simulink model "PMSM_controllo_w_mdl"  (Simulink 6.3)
settings: Solver=ode45  StartTime=0.0  StopTime=12.0  RelTol=1e-3
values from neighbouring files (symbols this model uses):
  bm = 0.8*N*metri*secondo/rad    (= 0.8)    [architetture_epicicloidale.m]    (also in architetture_epicicloidale_cont.m; architetture_epicicloidale_HEV.m; architetture_epicicloidale_prova.m; architetture_HEV_controllo.m)
  I_m = eye(m-1)    [architetture_epicicloidale.m]    (also in architetture_epicicloidale_cont.m; architetture_epicicloidale_HEV.m; architetture_epicicloidale_prova.m; architetture_HEV_controllo.m)
  Iw0 = 0*wI0    [architetture_epicicloidale.m]    (also in architetture_epicicloidale_cont.m = wI0; architetture_epicicloidale_HEV.m; architetture_epicicloidale_prova.m; architetture_HEV_controllo.m)
  Jm = 1.6*kg*metri^2    (= 1.6)    [architetture_epicicloidale.m]    (also in architetture_epicicloidale_cont.m; architetture_epicicloidale_HEV.m = 1.64945909552; architetture_epicicloidale_prova.m; architetture_HEV_controllo.m = 0.529459095518)
  Jr = Jr([1:m-1],[1:m-1])    [architetture_epicicloidale.m]    (also in architetture_epicicloidale_cont.m; architetture_epicicloidale_HEV.m; architetture_epicicloidale_prova.m; architetture_HEV_controllo.m)
  Kf = diag(diag(MLb)'./fliplr(tau_m(1:m-1)))    [architetture_epicicloidale_cont.m]    (also in architetture_epicicloidale_HEV.m; architetture_epicicloidale_prova.m; architetture_HEV_controllo.m; architetture_HEV_startstop.m)
  Kprop = 32.3*5    (= 161.5)    [architetture_HEV_controllo.m]    (also in architetture_HEV_startstop.m; PMSM_controllo_w.m = 32.3; architetture_HEV_startstop_1.m; architetture_HEV_startstop_2.m)
  Kr = Kr([1:m-1])    [architetture_epicicloidale.m]    (also in architetture_epicicloidale_cont.m; architetture_epicicloidale_HEV.m; architetture_epicicloidale_prova.m; architetture_HEV_controllo.m)
  Li = 0.1*Henry    (= 0.1)    [architetture_epicicloidale.m]    (also in architetture_epicicloidale_cont.m; architetture_epicicloidale_HEV.m; architetture_epicicloidale_prova.m; architetture_HEV_controllo.m)
  m = 5    [architetture_epicicloidale.m]    (also in architetture_epicicloidale_cont.m; architetture_epicicloidale_HEV.m; architetture_epicicloidale_prova.m; architetture_HEV_controllo.m)
  Mi = 0.08*Henry    (= 0.08)    [architetture_epicicloidale.m]    (also in architetture_epicicloidale_cont.m; architetture_epicicloidale_HEV.m; architetture_epicicloidale_prova.m; architetture_HEV_controllo.m)
  MKr = MKr([1:m-1],[1:m-1])    [architetture_epicicloidale.m]    (also in architetture_epicicloidale_cont.m; architetture_epicicloidale_HEV.m; architetture_epicicloidale_prova.m; architetture_HEV_controllo.m)
  MLb = MLb([1:m-1],[1:m-1])    [architetture_epicicloidale.m]    (also in architetture_epicicloidale_cont.m; architetture_epicicloidale_HEV.m; architetture_epicicloidale_prova.m; architetture_HEV_controllo.m)
  MR = MR([1:m-1],[1:m-1])    [architetture_epicicloidale.m]    (also in architetture_epicicloidale_cont.m; architetture_epicicloidale_HEV.m; architetture_epicicloidale_prova.m; architetture_HEV_controllo.m)
  Nar = 200    [architetture_epicicloidale.m]    (also in architetture_epicicloidale_cont.m; architetture_epicicloidale_HEV.m; architetture_epicicloidale_prova.m; architetture_HEV_controllo.m)
  Nc = 30    [architetture_epicicloidale.m]    (also in architetture_epicicloidale_cont.m; architetture_epicicloidale_HEV.m; architetture_epicicloidale_prova.m; architetture_HEV_controllo.m)
  p = 1    [architetture_epicicloidale.m]    (also in architetture_epicicloidale_cont.m; architetture_epicicloidale_HEV.m; architetture_epicicloidale_prova.m; architetture_HEV_controllo.m)
  Phir = 0.02*Weber    (= 0.02)    [architetture_epicicloidale.m]    (also in architetture_epicicloidale_cont.m; architetture_epicicloidale_HEV.m; architetture_epicicloidale_prova.m; architetture_HEV_controllo.m)
  Ri = 3*Ohm    (= 3)    [architetture_epicicloidale.m]    (also in architetture_epicicloidale_cont.m; architetture_epicicloidale_HEV.m; architetture_epicicloidale_prova.m; architetture_HEV_controllo.m = 0.1)
  Star = Si    [architetture_epicicloidale.m]    (also in architetture_epicicloidale_cont.m; architetture_epicicloidale_HEV.m; architetture_epicicloidale_prova.m; architetture_HEV_controllo.m)
  Tc = 0.05*ms    (= 5e-05)    [architetture_epicicloidale.m]    (also in architetture_epicicloidale_cont.m; architetture_epicicloidale_HEV.m; architetture_epicicloidale_prova.m; architetture_HEV_controllo.m)
  Tder = 0.0119*20    (= 0.238)    [architetture_HEV_controllo.m]    (also in architetture_HEV_startstop.m; PMSM_controllo_w.m; architetture_HEV_startstop_1.m; architetture_HEV_startstop_2.m)
  Thm0 = 0    [architetture_epicicloidale.m]    (also in architetture_epicicloidale_cont.m; architetture_epicicloidale_HEV.m; architetture_epicicloidale_prova.m; architetture_HEV_controllo.m)
  Tint = 0.2427*10    (= 2.427)    [architetture_HEV_controllo.m]    (also in architetture_HEV_startstop.m; PMSM_controllo_w.m = 0.2427; architetture_HEV_startstop_1.m; architetture_HEV_startstop_2.m)
  tTb = tTb(:,[1:m-1])    [architetture_epicicloidale.m]    (also in architetture_epicicloidale_cont.m; architetture_epicicloidale_HEV.m; architetture_epicicloidale_prova.m; architetture_HEV_controllo.m)
  Wm0 = 0*Wr_d    (= 0)    [architetture_epicicloidale.m]    (also in architetture_epicicloidale_cont.m = 62.5; architetture_epicicloidale_HEV.m; architetture_epicicloidale_prova.m; architetture_HEV_controllo.m)
libraries: simulink x2, POG_Sincronous_Motors x1

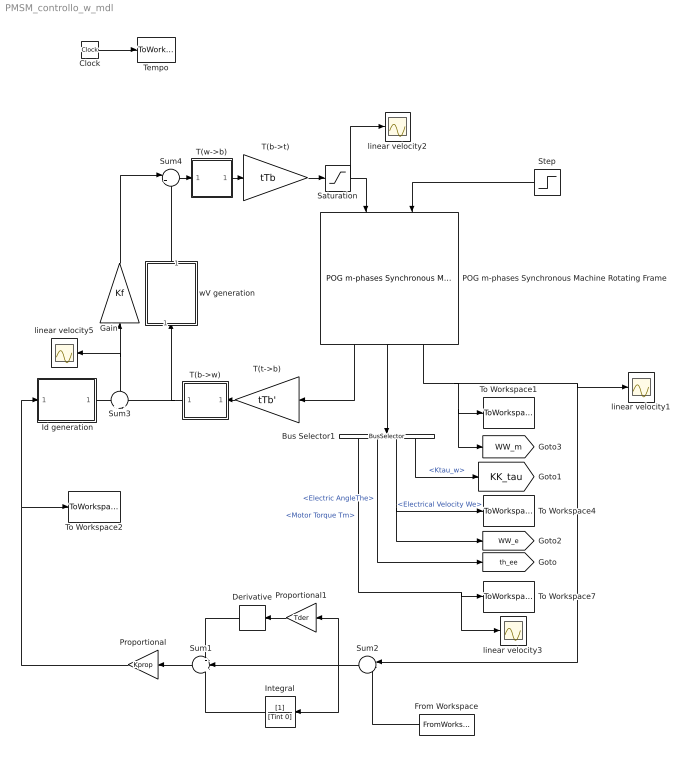
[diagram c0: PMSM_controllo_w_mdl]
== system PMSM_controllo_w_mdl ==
  " Id generation" : Subsystem
  Bus Selector1 : BusSelector  Orientation=down  OutputSignals=Motor Torque Tm,Electric AngleThe,Electrical Velocity We,Ktau_w
  Clock : Clock
  Derivative : Derivative  Orientation=left
  From Workspace : FromWorkspace  Orientation=left  VariableName=[T_in w_des]  SampleTime=0
  Gain : Gain  Orientation=up  Gain=Kf  Multiplication=Matrix(K*u) (u vector)
  Integral : TransferFcn  Orientation=left  Denominator=[Tint 0]
  POG m-phases Synchronous Machine Rotating Frame : POG_Sincronous_Motors/POG m-phases Synchronous Machine Rotating Frame  Orientation=down  Motor_Par=[m p]  Phase_Par=[Nc Star]  Electric_Par=[Ri Li Mi]  Mech_Par=[Jm bm]  Plux_Par=[Phir Nar]  Iniz_Cond=[Wm0; Thm0; Iw0]  TipoFlux=User defined  Tipo=Tipo  alfa=al  degree=6  TipoF=Tipo
  Proportional : Gain  Orientation=left  Gain=Kprop
  Proportional1 : Gain  Orientation=left  Gain=Tder
  Saturation : Saturate  UpperLimit=200  LowerLimit=-200
  Step : Step  Orientation=left  Time=5  After=100  SampleTime=0
  Sum1 : Sum  Orientation=left  Inputs=+++
  Sum2 : Sum  Orientation=left  Inputs=|-+
  Sum3 : Sum  Orientation=up  Inputs=+|-
  Sum4 : Sum  Inputs=|++
  T(b->t) : Gain  Gain=tTb  Multiplication=Matrix(K*u) (u vector)
  T(b->w) : Subsystem  Orientation=left  AncestorBlock=|
      | POG_Electric_Bloks/POG m-phases
      | Synchronous Machine
      | Rotating Frame/T(b->w)
  T(t->b) : Gain  Orientation=left  Gain=tTb'  Multiplication=Matrix(K*u) (u vector)
  T(w->b) : Subsystem  AncestorBlock=|
      | POG_Electric_Bloks/POG m-phases
      | Synchronous Machine
      | Rotating Frame/T(w->b)
  Tempo : ToWorkspace  VariableName=t  SampleTime=Tc  SaveFormat=Array
  To Workspace1 : ToWorkspace  VariableName=Wm  SampleTime=Tc  SaveFormat=Array
  To Workspace2 : ToWorkspace  VariableName=Tref  SampleTime=Tc  SaveFormat=Array
  To Workspace4 : ToWorkspace  VariableName=We  SampleTime=Tc  SaveFormat=Array
  To Workspace7 : ToWorkspace  VariableName=Tm  SampleTime=Tc  SaveFormat=Array
  linear velocity{1..3,5} (4 alike) : Scope
  wV generation : Subsystem  Orientation=up
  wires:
  Clock/1 -> Tempo/1
  POG m-phases Synchronous Machine Rotating Frame/3 -> To Workspace1/1, [WW_m], Sum2/1, linear velocity1/1
  POG m-phases Synchronous Machine Rotating Frame/2 -> Bus Selector1/1
  Bus Selector1/3 -> To Workspace4/1, [WW_e]  "<Electrical Velocity We>"
  T(w->b)/1(It) -> T(b->t)/1
  T(b->t)/1 -> Saturation/1
  T(t->b)/1 -> T(b->w)/1(Vt)
  T(b->w)/1(Vw) -> wV generation/1(In1), Sum3/2
  POG m-phases Synchronous Machine Rotating Frame/1 -> T(t->b)/1
  Bus Selector1/2 -> [th_ee]  "<Electric AngleThe>"
  Bus Selector1/1 -> To Workspace7/1, linear velocity3/1  "<Motor Torque Tm>"
  " Id generation"/1(Out1) -> Sum3/1
  Sum3/1 -> Gain/1, linear velocity5/1
  Sum4/1 -> T(w->b)/1(Iw)
  Gain/1 -> Sum4/1
  wV generation/1(Out1) -> Sum4/2
  Bus Selector1/4 -> [KK_tau]  "<Ktau_w>"
  Step/1 -> POG m-phases Synchronous Machine Rotating Frame/2
  Sum2/1 -> Integral/1, Proportional1/1, Sum1/2
  From Workspace/1 -> Sum2/2
  Sum1/1 -> Proportional/1
  Proportional1/1 -> Derivative/1
  Derivative/1 -> Sum1/1
  Integral/1 -> Sum1/3
  Proportional/1 -> " Id generation"/1(In1), To Workspace2/1
  Saturation/1 -> POG m-phases Synchronous Machine Rotating Frame/1, linear velocity2/1

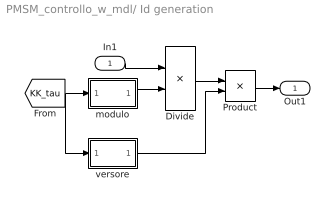
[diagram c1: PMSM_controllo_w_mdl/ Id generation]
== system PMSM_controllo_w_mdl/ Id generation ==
  In1 : Inport
  Divide : Product  Inputs=*/  OutScaling=2^-10
  Product : Product
  modulo : Subsystem
  versore : Subsystem
  Out1 : Outport
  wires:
  [KK_tau] -> modulo/1(In1), versore/1(In1)
  modulo/1(Out1) -> Divide/2
  Divide/1 -> Product/1
  versore/1(Out1) -> Product/2
  In1/1 -> Divide/1
  Product/1 -> Out1/1

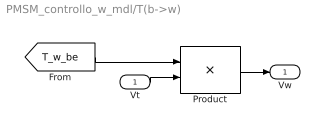
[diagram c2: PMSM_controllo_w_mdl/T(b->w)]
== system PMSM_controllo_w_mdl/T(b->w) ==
  Vt : Inport
  Product : Product  Multiplication=Matrix(*)
  Vw : Outport
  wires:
  Vt/1 -> Product/2
  Product/1 -> Vw/1
  [T_w_be] -> Product/1

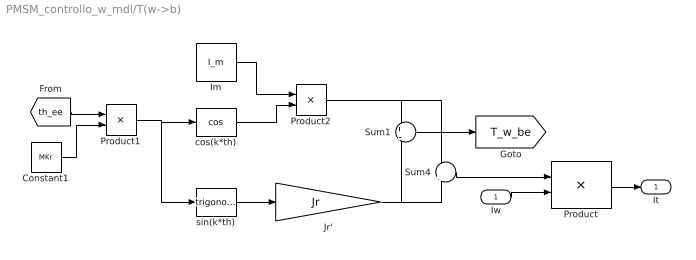
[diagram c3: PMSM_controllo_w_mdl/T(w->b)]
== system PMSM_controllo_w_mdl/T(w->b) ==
  Iw : Inport
  Constant1 : Constant  Value=MKr
  Im : Constant  Value=I_m  VectorParams1D=off
  Jr' : Gain  Gain=Jr  Multiplication=Matrix(K*u)
  Product : Product  Multiplication=Matrix(*)
  Product1 : Product
  Product2 : Product
  Sum1 : Sum  Inputs=+|-
  Sum4 : Sum  Inputs=+|+
  cos(k*th) : Trigonometry  Operator=cos
  sin(k*th) : Trigonometry
  It : Outport
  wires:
  Sum4/1 -> Product/1
  Product/1 -> It/1
  Iw/1 -> Product/2
  Jr'/1 -> Sum4/2, Sum1/2
  Product2/1 -> Sum4/1, Sum1/1
  Im/1 -> Product2/1
  cos(k*th)/1 -> Product2/2
  Product1/1 -> sin(k*th)/1, cos(k*th)/1
  Constant1/1 -> Product1/2
  [th_ee] -> Product1/1
  sin(k*th)/1 -> Jr'/1
  Sum1/1 -> [T_w_be]

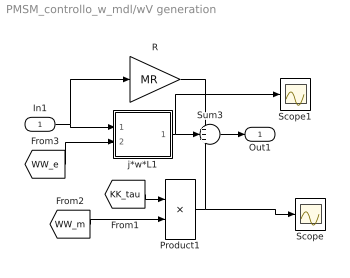
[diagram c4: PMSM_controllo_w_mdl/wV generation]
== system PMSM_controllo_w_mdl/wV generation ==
  In1 : Inport
  Product1 : Product  Multiplication=Matrix(*)
  R : Gain  Gain=MR  Multiplication=Matrix(K*u) (u vector)
  Scope : Scope
  Scope1 : Scope
  Sum3 : Sum  Inputs=+++
  j*w*L1 : Subsystem  AncestorBlock=|
      | POG_Electric_Bloks/POG m-phases
      | Synchronous Machine
      | Rotating Frame/j*w*L
  Out1 : Outport
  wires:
  [KK_tau] -> Product1/1
  [WW_m] -> Product1/2
  R/1 -> Sum3/1
  j*w*L1/1(Out1) -> Sum3/2, Scope1/1
  Product1/1 -> Sum3/3, Scope/1
  In1/1 -> j*w*L1/1(In1), R/1
  Sum3/1 -> Out1/1
  [WW_e] -> j*w*L1/2(In2)

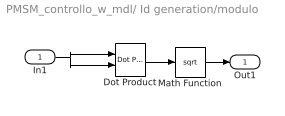
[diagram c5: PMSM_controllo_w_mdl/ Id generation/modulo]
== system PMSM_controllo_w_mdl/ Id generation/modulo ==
  In1 : Inport
  Dot Product : simulink/Math Operations/Dot Product  InputSameDT=on  OutDataType=sfix(16)  OutScaling=2^-10  DoSatur=off
  Math Function : Math  Operator=sqrt
  Out1 : Outport
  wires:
  In1/1 -> Dot Product/1, Dot Product/2
  Dot Product/1 -> Math Function/1
  Math Function/1 -> Out1/1

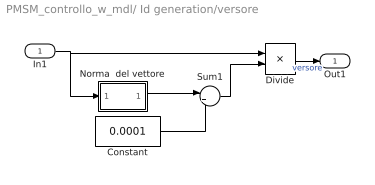
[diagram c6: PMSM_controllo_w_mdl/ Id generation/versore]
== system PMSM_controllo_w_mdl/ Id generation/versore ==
  In1 : Inport
  Constant : Constant  Value=0.0001
  Divide : Product  Inputs=*/  OutScaling=2^-10
  Norma  del vettore : Subsystem
  Sum1 : Sum  Inputs=|++
  Out1 : Outport
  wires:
  Divide/1 -> Out1/1  "versore"
  Constant/1 -> Sum1/2
  Sum1/1 -> Divide/2
  Norma  del vettore/1(Out1) -> Sum1/1
  In1/1 -> Norma  del vettore/1(In1), Divide/1

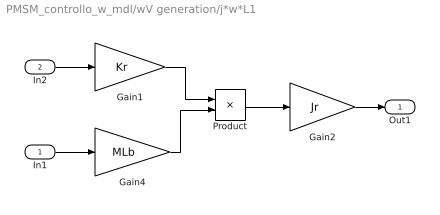
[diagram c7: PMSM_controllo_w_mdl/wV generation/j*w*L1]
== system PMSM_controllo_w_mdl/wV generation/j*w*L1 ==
  In1 : Inport
  In2 : Inport  Port=2
  Gain1 : Gain  Gain=Kr  Multiplication=Matrix(K*u) (u vector)
  Gain2 : Gain  Gain=Jr  Multiplication=Matrix(K*u) (u vector)
  Gain4 : Gain  Gain=MLb  Multiplication=Matrix(K*u) (u vector)
  Product : Product
  Out1 : Outport
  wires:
  In1/1 -> Gain4/1
  In2/1 -> Gain1/1
  Gain1/1 -> Product/1
  Gain4/1 -> Product/2
  Product/1 -> Gain2/1
  Gain2/1 -> Out1/1

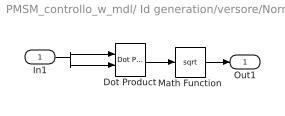
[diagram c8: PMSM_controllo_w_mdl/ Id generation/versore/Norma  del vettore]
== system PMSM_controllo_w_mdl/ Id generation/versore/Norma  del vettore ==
  In1 : Inport
  Dot Product : simulink/Math Operations/Dot Product  InputSameDT=on  OutDataType=sfix(16)  OutScaling=2^-10  DoSatur=off
  Math Function : Math  Operator=sqrt
  Out1 : Outport
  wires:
  Math Function/1 -> Out1/1
  Dot Product/1 -> Math Function/1
  In1/1 -> Dot Product/2, Dot Product/1
